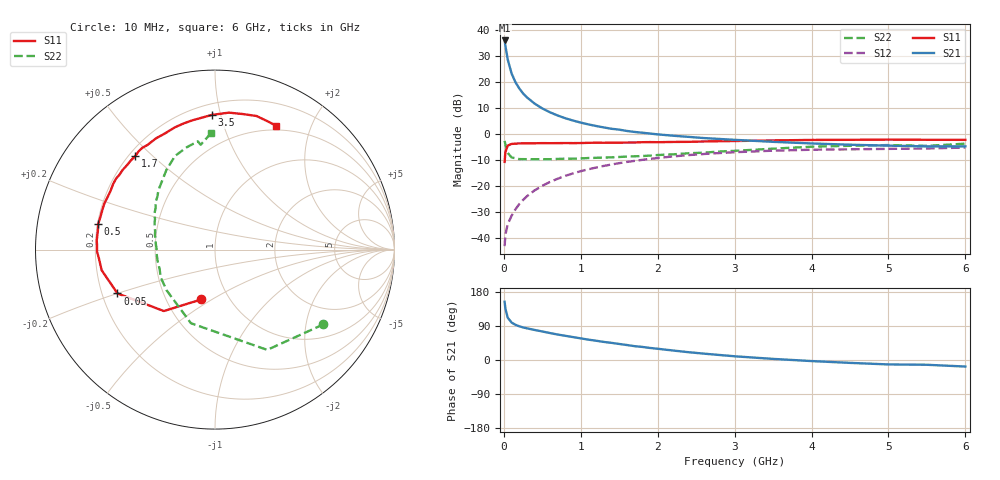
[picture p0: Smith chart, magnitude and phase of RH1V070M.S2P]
! SIEMENS Small Signal Semiconductors
! BFR106
! Si NPN RF Bipolar Junction Transistor in SOT23
! VCE = 1 V  IC = 70 mA
! Common Emitter S-Parameters:  August  1996
# GHz  S  MA  R  50
!  f  S11  S21  S12  S22
! GHz  MAG  ANG  MAG  ANG  MAG  ANG  MAG  ANG
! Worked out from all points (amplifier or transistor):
!   36 points, 10 MHz to 6 GHz, reference 50 ohm
!   highest |S21| = 36.1 dB at 10 MHz (marker M1)
!   |S21| within 3 dB of that: start of sweep to 25.8 MHz
!   unconditionally stable (mu >= 1): 131.2 MHz to end of sweep
!   at 250 MHz: K = 1.12, MAG = 18.5 dB, |S12| = -25.5 dB
!   at 1.4 GHz: K = 1.11, MAG = 4.8 dB, |S12| = -11.8 dB
!   at 6 GHz: K = 1.03, MAG = -0.8 dB, |S12| = -5.3 dB
!   S11 on the Smith chart (normalised r, x): 10 MHz: 0.74, -0.45; 50 MHz: 0.26, -0.20; 500 MHz: 0.20, +0.10; 1.7 GHz: 0.23, +0.44; 3.5 GHz: 0.27, +0.94; 6 GHz: 0.45, +1.52
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0.01  0.2885 -105.5  64.08 153.8  0.0068 70.1  0.7338 -34.6
0.02  0.4455 -129.8  51.08 135.9  0.0112 61.1  0.6298 -62.5
0.05  0.5957 -155.8  27.66 111.9  0.018 53.9  0.4316 -108.1
0.1  0.6419 -169.7  14.85 98.9  0.0262 60.0  0.3525 -139.7
0.15  0.6494 -176.1  10.05 92.9  0.0349 64.8  0.3398 -153.0
0.2  0.6574 -179.0  7.607 89.0  0.0441 67.8  0.3271 -160.5
0.25  0.6577 177.7  6.073 85.9  0.0531 69.4  0.3264 -166.2
0.3  0.6609 175.6  5.096 83.6  0.0627 70.5  0.326 -169.4
0.4  0.6608 171.1  3.863 79.3  0.0814 70.7  0.3257 -174.9
0.5  0.6662 167.6  3.11 75.3  0.0997 70.3  0.3256 -178.7
0.6  0.6639 163.7  2.622 71.1  0.1185 69.0  0.3257 178.5
0.7  0.6655 160.4  2.274 67.2  0.1366 67.9  0.3294 176.1
0.9  0.6661 154.1  1.816 60.4  0.1732 64.6  0.3332 170.8
1.1  0.6747 147.4  1.53 53.7  0.2081 61.2  0.343 167.2
1.3  0.6763 141.9  1.337 47.7  0.2416 57.3  0.3494 162.7
1.7  0.6844 130.6  1.095 36.5  0.302 49.9  0.3709 154.9
2.2  0.7016 117.9  0.925 25.0  0.3679 40.4  0.4035 145.2
2.8  0.724 104.1  0.802 13.3  0.4276 29.6  0.4575 133.5
3.5  0.7504 91.4  0.705 2.9  0.476 18.3  0.5203 121.3
4.5  0.7714 78.0  0.62 -7.6  0.5056 4.7  0.5914 105.5
5.5  0.7724 67.4  0.576 -12.6  0.5248 -3.1  0.5894 97.8
6  0.7694 63.7  0.577 -17.3  0.5462 -9.5  0.6504 91.8
